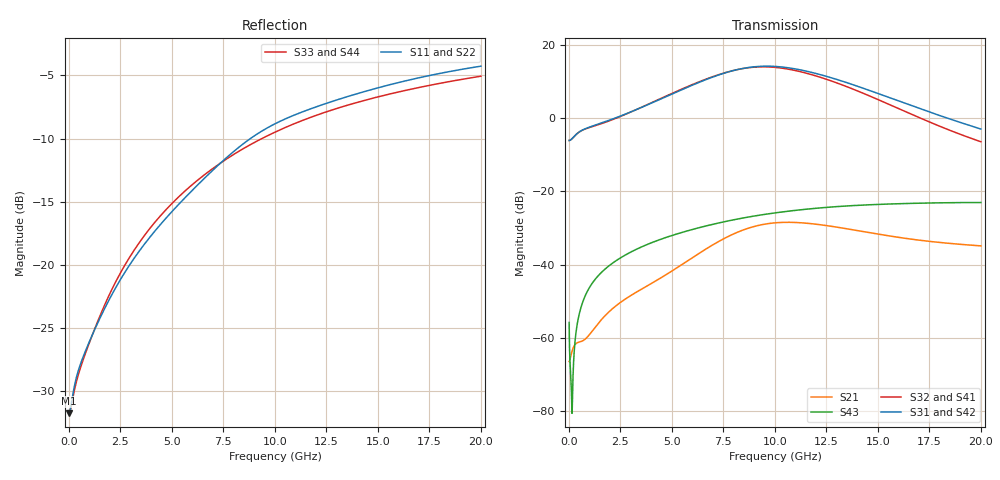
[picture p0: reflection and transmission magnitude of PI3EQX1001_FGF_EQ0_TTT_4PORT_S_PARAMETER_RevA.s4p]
! NPort=4 DATA=2000 NOISE=0 GROUPDELAY=0 COMPLEX_DATAFORMAT=POLAR
! NumOfBlock=1 NumOfParam=0
! .MODEL Smodel S TSTONEFILE=PI3EQX1002B_FGF_EQ0_TTT_4PORT_S_PARAMETER_RevA.s4p TYPE=S
!  -- The above .MODEL line can be used for the S element in the netlist.
! The s parameter is extracted from the linear redriver, it is not bi-directional; only s(4,1)s(4,2) and s(3,1)s(3,2)
! should be the insertion loss
!Port definition:
!Port1 = input+
!Port2 = input¨C
!Port3 = output+
!Port4 = output-
# Hz S MA R  50
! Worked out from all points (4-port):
!   2000 points, 10 MHz to 20 GHz, reference 50 ohm
!   strongest paths, dB at 10 MHz, 5.01 GHz, 10.01 GHz, 15.01 GHz, 20 GHz:
!     S31: -6.1, 6.6, 14.1, 6.7, -3.0
!     S42: -6.1, 6.6, 14.1, 6.7, -3.0
!     S32: -6.1, 6.8, 13.9, 5.1, -6.4
!     S41: -6.1, 6.7, 13.8, 5.0, -6.5
!     S43: -55.8, -32.0, -25.9, -23.5, -23.0
!     S21: -66.4, -41.7, -28.6, -31.7, -34.9
!   lowest |S11| = -31.7 dB at 10 MHz (marker M1), VSWR 1.05, Z = 47.5 - j0.063 ohm
!   |S11| at or under -10 dB: start of sweep to 8.812 GHz
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1e7  0.02591 -178.5  0.0004922 2.7  3.669e-05 -0.2  4.787e-05 -0.1
     0.0004763 2.9  0.02597 -178.7  4.577e-05 -0.2  5.994e-05 -0.1
     0.4961 0.1  0.496 -179.9  0.02616 178.4  0.001615 -59.2
     0.4958 -179.9  0.4959 0.1  0.001626 -58.9  0.02612 178.4
6.54e9  0.2187 -104.9  0.01495 95.5  2.253e-05 -30.9  3.255e-05 -29.4
        0.01564 93.8  0.217 -104.9  2.965e-05 -26.3  4.115e-05 -24.7
        3.261 -51.8  3.312 131.8  0.226 -111.4  0.03317 59.0
        3.302 131.7  3.256 -51.7  0.03316 59.0  0.226 -111.4
8.59e9  0.3068 -107.3  0.02959 65.9  2.014e-05 -28.1  3.195e-05 -31.8
        0.03067 64.5  0.3049 -107.3  2.972e-05 -25.8  3.881e-05 -24.4
        4.848 -110.6  4.821 73.1  0.2923 -113.9  0.04416 46.6
        4.801 73.1  4.844 -110.4  0.04408 46.5  0.2921 -113.9
1.047e10  0.377 -112.8  0.0366 29.6  2.186e-05 -22.7  3.313e-05 -40.4
          0.03784 28.4  0.3742 -112.9  3.142e-05 -33.6  4.022e-05 -23.7
          4.942 -172.4  4.753 11.6  0.3487 -116.9  0.05313 34.2
          4.73 11.7  4.939 -172.2  0.05295 34.2  0.3485 -116.9
1.296e10  0.4482 -118.4  0.03161 -5.6  2.841e-05 -36.7  3.044e-05 -60.9
          0.0327 -6.7  0.4444 -118.5  2.88e-05 -52.4  4.577e-05 -34.1
          3.404 115.9  3.058 -59.0  0.4148 -121.1  0.06205 17.7
          3.04 -58.8  3.402 116.0  0.0619 17.8  0.4147 -121.1
1.554e10  0.5152 -123.1  0.02382 -23.5  2.823e-05 -68.5  2.267e-05 -89.1
          0.02472 -24.6  0.5109 -123.2  2.068e-05 -77.0  4.296e-05 -56.1
          1.913 58.1  1.541 -113.5  0.4736 -125.1  0.06735 1.7
          1.531 -113.1  1.911 58.3  0.06729 1.8  0.4732 -125.0
2e10  0.6111 -130.8  0.01742 -32.7  1.43e-05 -150.9  1.178e-05 150.1
      0.01805 -34.5  0.6057 -130.9  7.614e-06 134.0  1.699e-05 -95.8
      0.7096 -13.0  0.4763 -167.4  0.5577 -131.1  0.07054 -23.3
      0.4742 -166.6  0.7083 -12.9  0.07052 -23.4  0.5576 -131.1
